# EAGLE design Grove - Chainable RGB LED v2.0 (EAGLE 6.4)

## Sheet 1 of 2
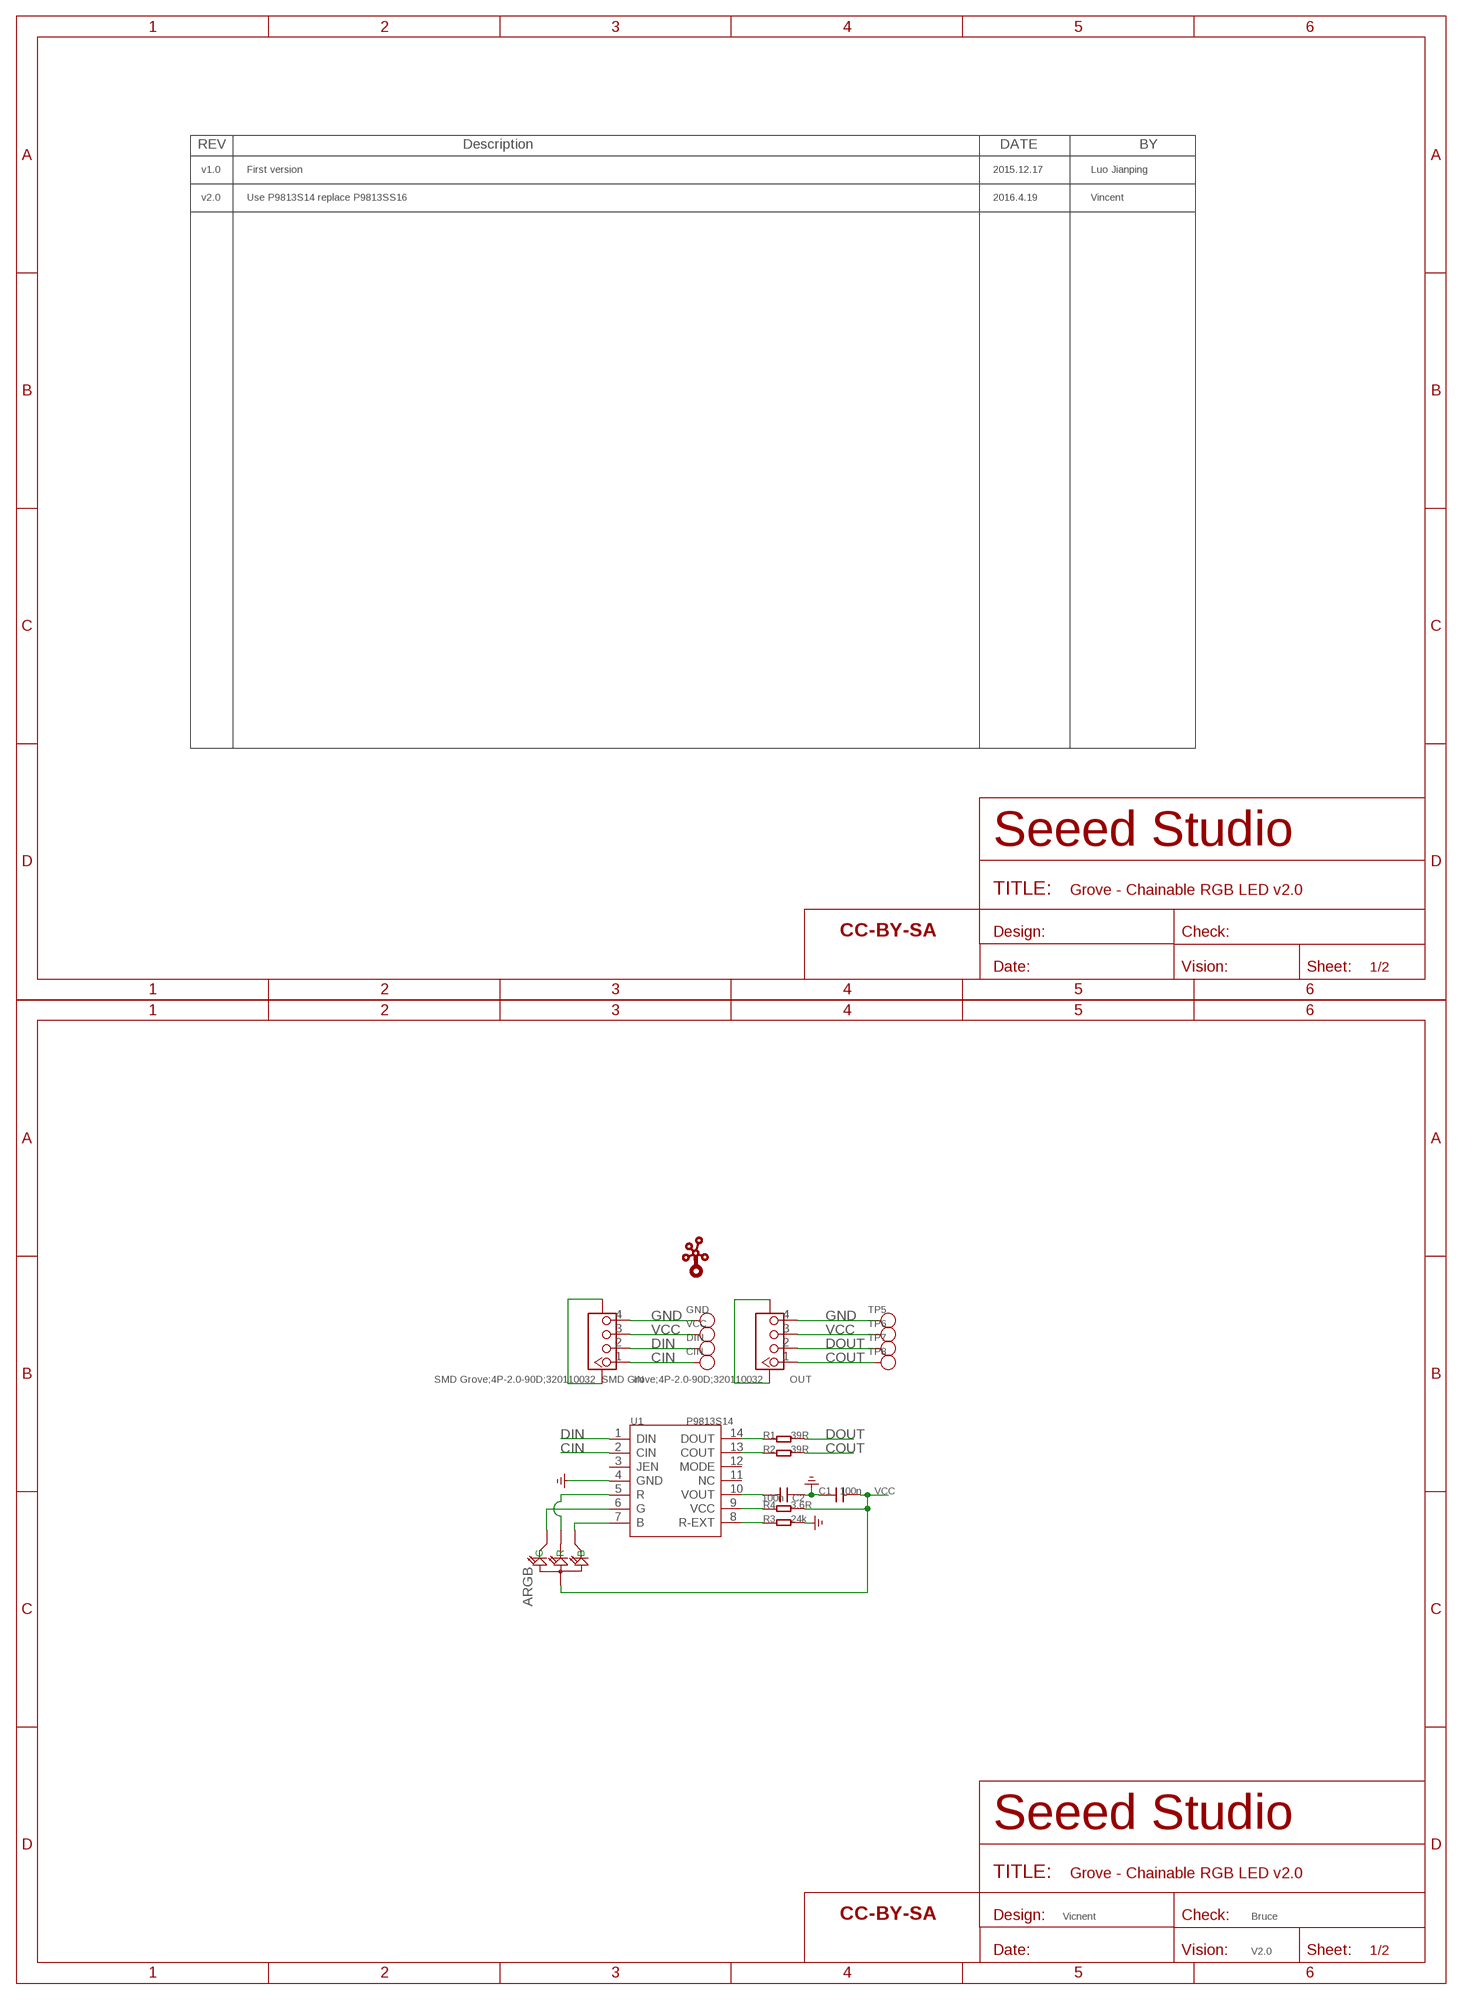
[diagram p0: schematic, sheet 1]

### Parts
ARGB  LED-ARGB-DIP2.0  [ARGB/2.0]
C1  100n  C-0603  [0603]
C2  100n  C-0603  [0603]
CIN  TEST-POINT'4545'  [TP-D45MIL]
DIN  TEST-POINT'4545'  [TP-D45MIL]
FR1  SEEEDSTUDIO-OPEN-SCH-FRAME  [SEEEDSTUDIO-PCB-FRAME]
FR2  SEEEDSTUDIO-OPEN-SCH-FRAME  [SEEEDSTUDIO-PCB-FRAME]
GND  TEST-POINT'4545'  [TP-D45MIL]
IN  SMD Grove;4P-2.0-90D;320110032  GROVE-CONNECTOR-SMD'90D'  [HW4-SMD-2.0-90D]
OUT  SMD Grove;4P-2.0-90D;320110032  GROVE-CONNECTOR-SMD'90D'  [HW4-SMD-2.0-90D]
R1  39R  R-0603  [0603]
R2  39R  R-0603  [0603]
R3  24k  R-0603  [0603]
R4  3.6R  R-0603  [0603]
TP5  TEST-POINT'4545'  [TP-D45MIL]
TP6  TEST-POINT'4545'  [TP-D45MIL]
TP7  TEST-POINT'4545'  [TP-D45MIL]
TP8  TEST-POINT'4545'  [TP-D45MIL]
U1  P9813S14  DRIVER-P9813-SOP14  [SOP14-1.27-8.65X3.9X1.35MM]
U$1  TWIGLOGOTWIGLOGO_SMALL  [TWIGLOGO_SMALL]
VCC  TEST-POINT'4545'  [TP-D45MIL]

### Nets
CIN: CIN.T IN.1 U1.2(CIN)
COUT: OUT.1 R2.2 TP8.T
DIN: DIN.T IN.2 U1.1(DIN)
DOUT: OUT.2 R1.2 TP7.T
GND: C1.1 C2.1 GND.T IN.4 IN.SS1 IN.SS2 OUT.4 OUT.SS1 OUT.SS2 R3.2 TP5.T U1.4(GND) ; supply symbol labelled GND_POWER
N$1: ARGB.4(B) U1.7(B)
N$2: ARGB.3(G) U1.6(G)
N$3: ARGB.1(R) U1.5(R)
N$4: R1.1 U1.14(DOUT)
N$5: R2.1 U1.13(COUT)
N$6: R3.1 U1.8(R-EXT)
N$8: C2.2 U1.10(VOUT)
N$9: R4.1 U1.9(VCC)
VCC: ARGB.2(+) C1.2 IN.3 OUT.3 R4.2 TP6.T VCC.T
Unconnected: U1.3(JEN) U1.11(NC) U1.12(MODE)

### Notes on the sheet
- v1.0 | First version | 2015.12.17 | Luo Jianping
- v2.0 | Use P9813S14 replace P9813SS16 | 2016.4.19 | Vincent
- Vicnent | Bruce
- V2.0

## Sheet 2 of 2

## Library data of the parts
ARGB = Discrete:LED-ARGB*
C1 C2 = Discrete:C*: Ceramic Capacitors
CIN DIN GND TP5-TP8 VCC = Discrete-new:TEST-POINT; PARTNO: DNP
FR1 FR2 = moudle-new:SEEEDSTUDIO-OPEN-SCH-FRAME
IN OUT = Connector-new:GROVE-CONNECTOR-SMD: 4P-SMD-2.0:320110030;4P-SMD-2.0-90D:320110032
R1-R4 = Discrete:R*
U1 = IC-new:DRIVER-P9813-SOP14
U$1 = seeedleo:TWIGLOGO

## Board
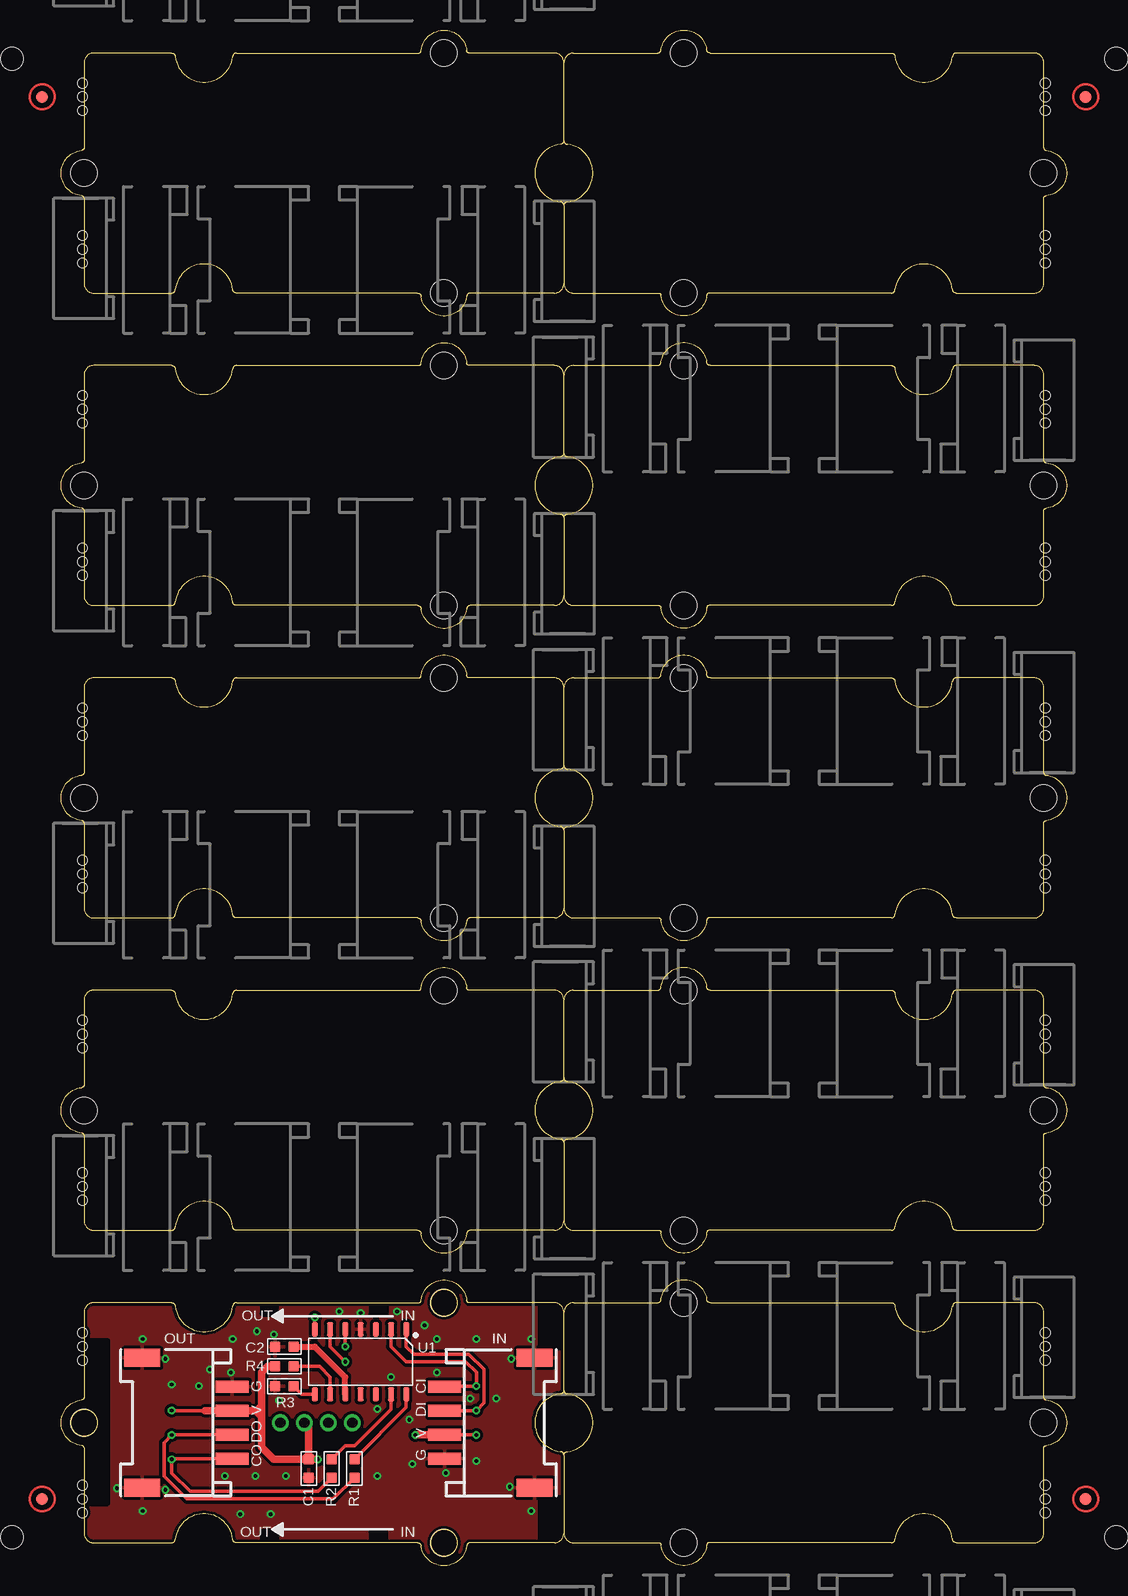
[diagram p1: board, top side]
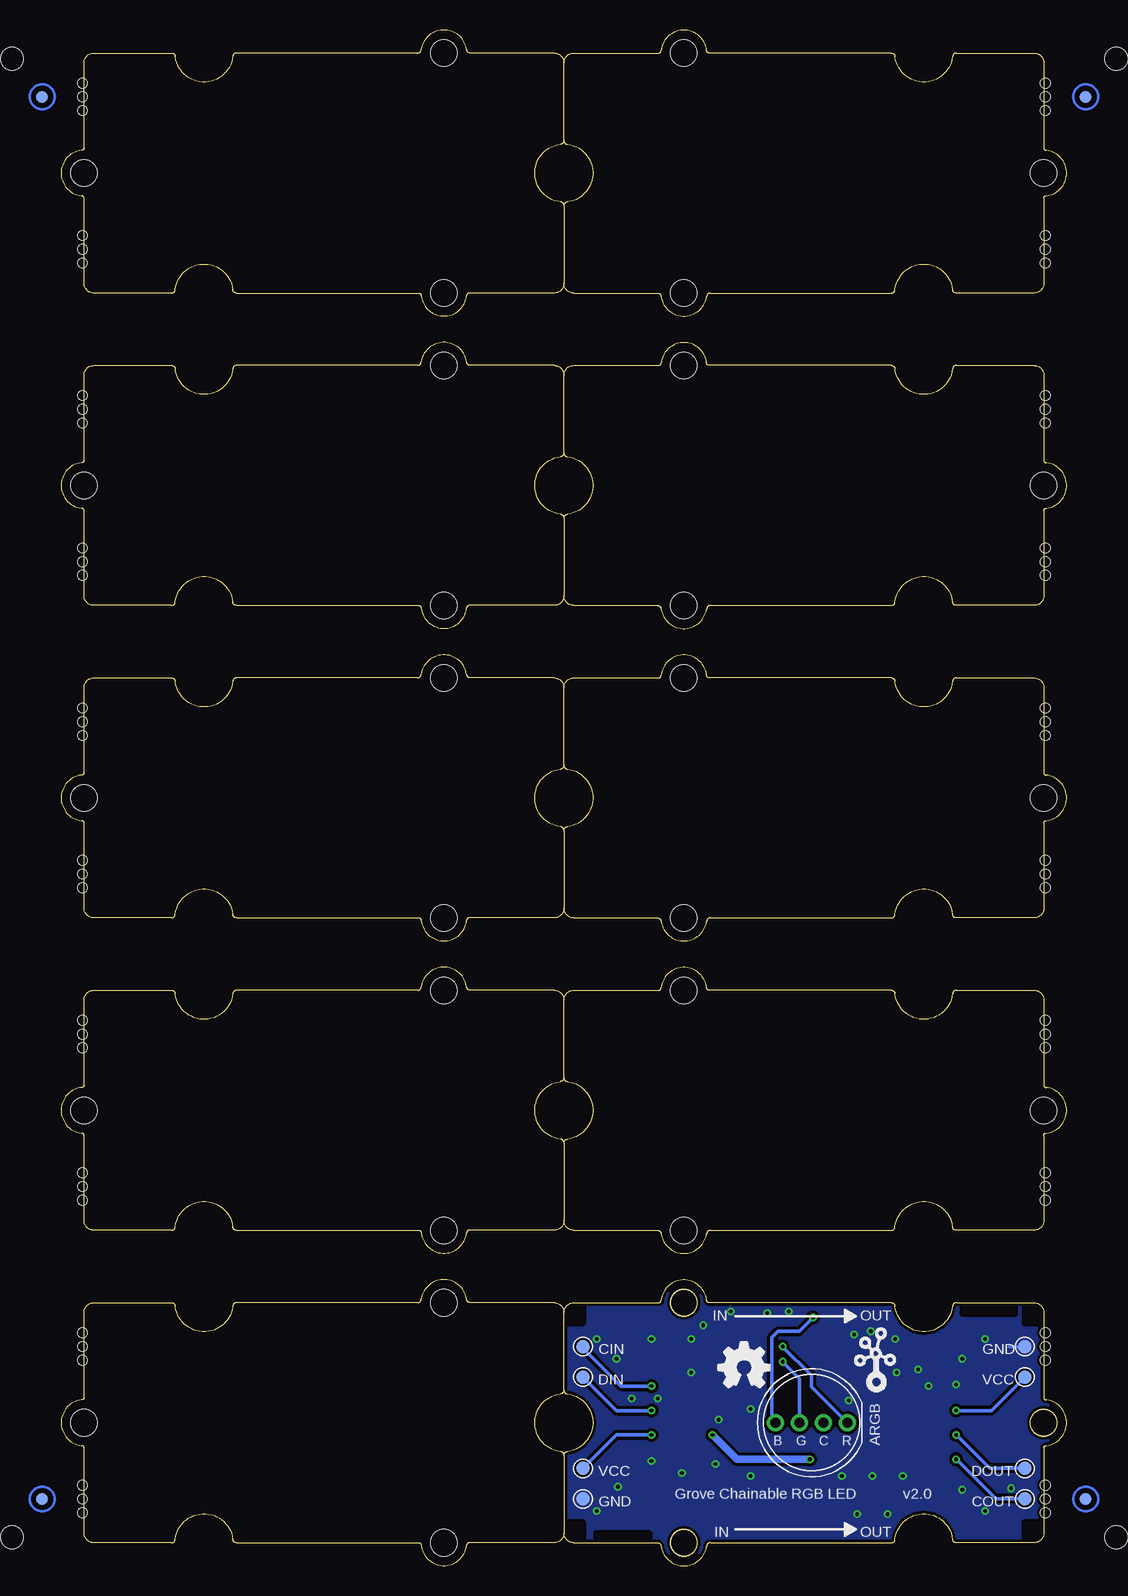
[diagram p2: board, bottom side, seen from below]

Size 83.82 x 127.98 mm. Coordinates in mm from the lower left corner, seen from the top.
Copper layers (1*16): Top 0.035mm / dielectric 1.5mm / Bottom 0.035mm
Design rules "SeeedStudio_2layer_DRU_no_angle_20140221 *": minimum track width 6mil, minimum drill 12mil, track to track 6mil, track to pad 6mil, pad to pad 6mil, via to via 6mil, smd to smd 0mil, copper to edge 10mil, drill to drill 10mil, minimum pad ring 10mil, minimum via ring 6mil, stop-mask expansion 2mil, vias tented up to drill 25mil, thermal gap 10mil
Holes 0.8 mm at 1.78,17.13 1.78,19.41 1.78,18.27 1.78,4.43 1.78,6.71 1.78,5.57 82.04,4.43 82.04,6.71 82.04,5.57 82.04,17.13 82.04,19.41 82.04,18.27 82.04,30.46 82.04,32.75 82.04,31.61 82.04,43.16 82.04,45.45 82.04,44.31 82.04,56.5 82.04,58.78 82.04,57.64 82.04,69.2 82.04,71.48 82.04,70.34 82.04,82.53 82.04,84.82 82.04,83.68 82.04,95.23 82.04,97.52 82.04,96.38 82.04,108.57 82.04,110.85 82.04,109.71 82.04,121.27 82.04,123.55 82.04,122.41 1.78,32.75 1.78,30.46 1.78,31.61 1.78,45.45 1.78,43.16 1.78,44.31 1.78,58.78 1.78,56.5 1.78,57.64 1.78,71.48 1.78,69.2 1.78,70.34 1.78,84.82 1.78,82.53 1.78,83.68 1.78,97.52 1.78,95.23 1.78,96.38 1.78,110.85 1.78,108.57 1.78,109.71 1.78,123.55 1.78,121.27 1.78,122.41
Holes 1.91 mm at 87.95,125.59 -4.13,125.59 -4.13,2.4 87.95,2.4

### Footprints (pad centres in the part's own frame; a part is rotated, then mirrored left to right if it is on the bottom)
ARGB/2.0 = drill 0.85 pad 1.4: 1 3,0; 2 1,0; 3 -1,0; 4 -3,0
0603 = smd 0.889 x 0.889: 1 -0.762,0; 2 0.762,0
TP-D45MIL = smd 1.143 x 1.143: T 0,0
HW4-SMD-2.0-90D = smd 1.01 x 2.74: 1 -3,-0.1; 2 -1,-0.1; 3 1,-0.1; 4 3,-0.1 | smd 1.5 x 3: SS1 -5.4,7.4; SS2 5.4,7.4
ROUND-MARK-1.0 = smd 1.016 x 1.016: P$1 0,0
SOP14-1.27-8.65X3.9X1.35MM = smd 0.525 x 1.2: 1 -3.81,-2.7; 2 -2.54,-2.7; 3 -1.27,-2.7; 4 0,-2.7; 5 1.27,-2.7; 6 2.54,-2.7; 7 3.81,-2.7; 8 3.81,2.7; 9 2.54,2.7; 10 1.27,2.7; 11 0,2.7; 12 -1.27,2.7; 13 -2.54,2.7; 14 -3.81,2.7
GROVE-TEST-PLATFORM = hole 2.2: -10,-10; -10,10; 20,0
GROVE-1*2-TEST-PLATFORM-BOTTOM = hole 2.2: 10.635,10; 10.635,-10; -19.365,0

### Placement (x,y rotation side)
ARGB  21.27,11.92 0 bottom
C1  20.64,8.11 90 top
C2  18.61,18.27 0 top
CIN  40.32,18.27 0 bottom
DIN  40.32,15.73 0 bottom
FR1  not placed on the board
FR2  not placed on the board
GND  40.32,5.57 0 bottom
IN  32.07,11.92 270 top
OUT  14.16,11.92 90 top
P1  [ROUND-MARK-1.0]  85.41,122.41 180 top
P2  [ROUND-MARK-1.0]  -1.59,122.41 180 top
P3  [ROUND-MARK-1.0]  85.41,5.57 180 top
P4  [ROUND-MARK-1.0]  -1.59,5.57 180 top
P5  [ROUND-MARK-1.0]  85.41,122.41 180 bottom
P6  [ROUND-MARK-1.0]  -1.59,122.41 180 bottom
P7  [ROUND-MARK-1.0]  -1.59,5.57 180 bottom
P8  [ROUND-MARK-1.0]  85.41,5.57 180 bottom
R1  24.45,8.11 270 top
R2  22.54,8.11 270 top
R3  18.61,14.97 180 top
R4  18.61,16.62 180 top
TP5  3.49,18.27 0 bottom
TP6  3.49,15.73 0 bottom
TP7  3.49,8.11 0 bottom
TP8  3.49,5.57 0 bottom
U1  24.96,17 180 top
U2  [GROVE-TEST-PLATFORM]  21.91,90.03 180 top
U3  [GROVE-TEST-PLATFORM]  61.91,90.03 0 top
U4  [GROVE-TEST-PLATFORM]  21.91,63.99 180 top
U5  [GROVE-TEST-PLATFORM]  61.91,63.99 0 top
U6  [GROVE-TEST-PLATFORM]  21.91,37.96 180 top
U7  [GROVE-TEST-PLATFORM]  61.91,37.96 0 top
U8  [GROVE-TEST-PLATFORM]  61.91,11.92 0 top
U10  [GROVE-TEST-PLATFORM]  21.91,116.06 180 top
U11  [GROVE-TEST-PLATFORM]  61.91,116.06 0 top
U$1  18.1,14.33 0 bottom
U$3  [GROVE-1*2-TEST-PLATFORM-BOTTOM]  21.27,11.92 0 top
U$8  [OSHW_FILLX150_NOTEXT]  29.02,14.84 0 bottom
VCC  40.32,8.11 0 bottom

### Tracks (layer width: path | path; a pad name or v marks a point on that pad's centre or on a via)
CIN  (via drill 0.3 pad 0.64)
  Top 0.305: IN.1 32.02,14.97 v34.61,14.97 34.61,16.11 33.72,17 28.77,17 27.5,18.27 U1.2
  Bottom 0.305: CIN.T 40.32,18.14 37.15,14.97 v34.61,14.97
COUT  (via drill 0.3 pad 0.64)
  Top 0.305: 12.72,8.92 OUT.1 9.26,8.92 v9.21,8.87 9.21,7.73 10.73,6.21 21.4,6.21 R2.2
  Bottom 0.305: TP8.T 5.91,5.57 v9.21,8.87
DIN  (via drill 0.3 pad 0.64)
  Top 0.305: IN.2 31.98,12.94 v34.61,12.94 35.24,13.57 35.24,16.37 33.97,17.64 29.4,17.64 28.77,18.27 U1.1
  Bottom 0.305: DIN.T 37.53,12.94 v34.61,12.94
DOUT  (via drill 0.3 pad 0.64)
  Top 0.305: R1.2 22.67,5.57 10.48,5.57 8.57,7.48 8.57,10.27 v9.21,10.91 9.22,10.92 OUT.2
  Bottom 0.305: TP7.T 6.41,8.11 v9.21,10.91
GND  (via drill 0.3 pad 0.64)
  Bottom 0.305: TP5.T 4.76,18.27
  other vias: 18.16,13.76 16.32,19.54 18.73,7.48 16.19,7.48 13.65,7.48 14.29,18.91 12.38,16.37 9.21,15.1 31.31,16.11 29.02,12.18 29.27,8.49 26.35,7.48 34.61,8.75 27.5,15.73 31.31,18.91 34.61,18.91 14.92,4.3 17.46,4.3 23.18,21.19 17.72,19.29 37.53,17.26 37.4,6.59 8.7,17.26 8.7,6.33 30.29,20.05 28,21.19 24.96,21.07 26.35,13.06 32.07,7.73 11.49,14.97 14.16,16.11 6.8,4.56 39.18,18.91 36.26,13.95 34.1,13.95 39.18,4.56 4.64,6.46 6.8,18.91
  pour Bottom (isolate 0.254): 1.59,22.72 42.23,22.72 42.23,1.13 1.59,1.13
  pour Top (isolate 0.254): 1.59,22.72 42.23,22.72 42.23,1.13 1.59,1.13
N$1  (via drill 0.3 pad 0.64)
  Top 0.305: U1.7 v21.15,20.68
  Bottom 0.305: ARGB.4 24.32,11.92 24.58,12.18 24.58,19.03 24.07,19.54 22.29,19.54 v21.15,20.68
N$2  (via drill 0.3 pad 0.64)
  Top 0.305: U1.6 22.42,18.27 v23.69,17
  Bottom 0.305: ARGB.3 22.27,15.59 v23.69,17
N$3  (via drill 0.3 pad 0.64)
  Top 0.305: U1.5 v23.69,18.27
  Bottom 0.305: ARGB.1 21.27,14.92 21.27,15.86 v23.69,18.27
N$4
  Top 0.305: R1.1 28.77,13.19 U1.14
N$5
  Top 0.305: R2.1 23.69,10.02 24.45,10.02 27.5,13.06 U1.13
N$6
  Top 0.305: U1.8 20.04,14.3 R3.1
N$8
  Top 0.508: U1.10 23.69,15.73 21.15,18.27 C2.2
N$9
  Top 0.305: U1.9 22.42,15.73 21.53,16.62 R4.1
VCC  (via drill 0.3 pad 0.64)
  Top 0.305: v34.61,10.91 31.98,10.91 IN.3 | v9.21,12.94 11.99,12.94 12,12.92
  Top 0.61: C1.2 20.64,11.56 ARGB.2 | 12,12.92 OUT.3 15.96,12.92 16.21,12.92 | C1.2 v21.4,8.87 | v29.53,10.91 31.95,10.91 IN.3 | C1.2 17.72,8.87 16.7,9.89 16.7,12.43 | R4.2 17.21,16.62 16.7,16.11 16.7,13.32 | 16.7,12.43 16.7,12.94 | 16.7,12.94 16.7,13.32 | 16.3,12.92 16.69,12.92 16.7,12.94 | 16.21,12.92 16.3,12.92 | 16.3,12.92 16.7,13.32 | 16.21,12.92 16.7,12.43
  Bottom 0.305: VCC.T 37.53,10.91 v34.61,10.91 | TP6.T 6.29,12.94 v9.21,12.94
  Bottom 0.61: v21.4,8.87 27.5,8.87 v29.53,10.91

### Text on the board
tPlace: OUT | IN | G | CI | V | DI | DO | V | G | CO | OUT | IN
bPlace: OUT | IN | GND | VCC | DOUT | COUT | v2.0 | Grove Chainable RGB LED | OUT | IN

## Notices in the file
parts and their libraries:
moudle-new: This work is licensed under the Creative Commons Attribution 4.0 International License.
To view a copy of this license,visit:
http://creativecommons.org/licenses/by-sa/4.0
moudle-new: CC-BY-SA
